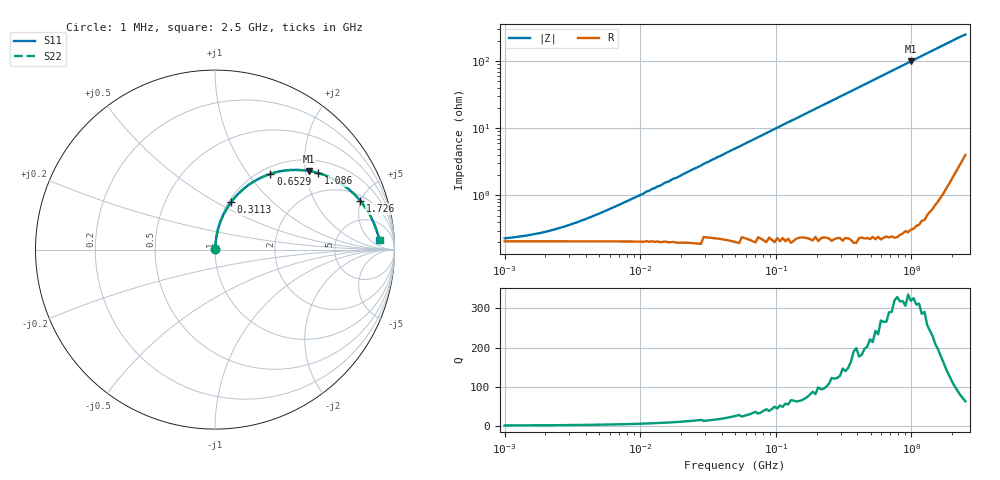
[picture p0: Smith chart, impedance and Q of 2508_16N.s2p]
# MHz S MA R 50
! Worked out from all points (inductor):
!   170 points, 1 MHz to 2.5 GHz, reference 50 ohm
!   read as one part in series: L = 15.9 nH near 6.372 MHz
!   highest Q = 326 at 990.4 MHz (marker M1), where L = 16 nH
!   S11 on the Smith chart (normalised r, x): 1 MHz: 1.00, +0.00; 311.3 MHz: 1.03, +0.59; 652.9 MHz: 1.11, +1.29; 1.086 GHz: 1.35, +2.36; 1.726 GHz: 2.46, +4.94; 2.5 GHz: 16, +10
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1  0.002345 23.4  0.998 -0.1  0.998 -0.1  0.002345 23.4
2.003  0.002851 40.9  0.998 -0.1  0.998 -0.1  0.002852 40.9
3.829  0.004176 58.8  0.998 -0.2  0.998 -0.2  0.004178 58.8
10.603  0.01 77.1  0.998 -0.6  0.998 -0.6  0.01 77.1
11.105  0.011 77.6  0.998 -0.7  0.998 -0.7  0.011 77.6
11.631  0.011 78.1  0.998 -0.7  0.998 -0.7  0.011 78.1
12.182  0.012 78.6  0.998 -0.7  0.998 -0.7  0.012 78.6
13.998  0.013 79.8  0.998 -0.8  0.998 -0.8  0.013 79.8
15.355  0.015 80.6  0.998 -0.9  0.998 -0.9  0.015 80.6
18.479  0.017 81.8  0.998 -1.1  0.998 -1.1  0.017 81.8
51.171  0.048 84.3  0.997 -3.1  0.997 -3.1  0.048 84.3
102.474  0.095 82.5  0.993 -6.2  0.993 -6.2  0.095 82.5
187.066  0.172 78.1  0.983 -11.2  0.983 -11.2  0.172 78.1
311.289  0.28 71.2  0.958 -18.4  0.958 -18.4  0.28 71.2
450.829  0.389 63.7  0.919 -26.0  0.919 -26.0  0.389 63.7
652.922  0.523 53.8  0.85 -36.0  0.85 -36.0  0.523 53.8
683.861  0.541 52.4  0.839 -37.4  0.839 -37.4  0.541 52.4
990.414  0.683 39.9  0.728 -49.9  0.728 -49.9  0.683 39.9
1086.499  0.716 36.5  0.695 -53.3  0.695 -53.3  0.717 36.5
1369.494  0.792 27.7  0.606 -62.1  0.606 -62.1  0.793 27.7
1726.199  0.854 18.6  0.515 -71.1  0.515 -71.1  0.854 18.6
2500  0.917 3.2  0.382 -85.8  0.382 -85.8  0.918 3.2
